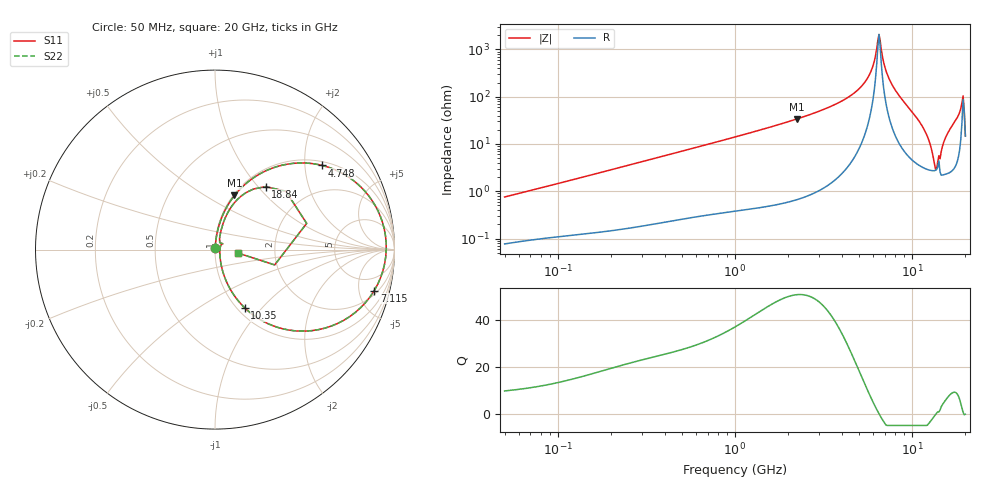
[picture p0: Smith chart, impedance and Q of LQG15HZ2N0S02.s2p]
!Murata Part Number: LQG15HZ2N0S02
!These Parameters are Measured in Series Mode Connection
!  o--[Z]--o
!Port1  Port2
!  o-------o
!Freq. Start=50[MHz] Stop=20[GHz], 401[Steps]
# Hz S RI R 50
!Freq.(Hz) S11(Real) S11(Imag) S21(Real) S21(Imag) S12(Real) S12(Imag) S22(Real) S22(Imag)
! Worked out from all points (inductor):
!   401 points, 50 MHz to 20 GHz, reference 50 ohm
!   read as one part in series: L = 2.36 nH near 51.52 MHz
!   highest Q = 51.1 at 2.245 GHz (marker M1), where L = 2.41 nH
!   self-resonance near 6.503 GHz
!   S11 on the Smith chart (normalised r, x): 50 MHz: 1.00, +0.02; 4.748 GHz: 1.11, +2.45; 7.115 GHz: 2.47, -7.03; 10.35 GHz: 1.08, -0.81; 18.84 GHz: 1.25, +1.10; 20 GHz: 1.29, -0.05
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5e7  0.000824 0.00751  0.9992 -0.00751  0.9992 -0.00751  0.000824 0.00751
1.364002e8  0.00161 0.0196  0.9984 -0.0196  0.9984 -0.0196  0.00161 0.0196
3.721004e8  0.00483 0.0521  0.9952 -0.0521  0.9952 -0.0521  0.00483 0.0521
1e9  0.0229 0.1369  0.9771 -0.1369  0.9771 -0.1369  0.0229 0.1369
2.245319e9  0.1085 0.3014  0.8915 -0.3014  0.8915 -0.3014  0.1085 0.3014
2.728004e9  0.1647 0.3611  0.8353 -0.3611  0.8353 -0.3611  0.1647 0.3611
3.680849e9  0.3263 0.4564  0.6737 -0.4564  0.6737 -0.4564  0.3263 0.4564
4.748272e9  0.597 0.4689  0.403 -0.4689  0.403 -0.4689  0.597 0.4689
5.769027e9  0.8744 0.2746  0.1256 -0.2746  0.1256 -0.2746  0.8744 0.2746
6.503449e9  0.9541 0.00111  0.0459 -0.00111  0.0459 -0.00111  0.9541 0.00111
7.114996e9  0.8871 -0.2287  0.1129 0.2287  0.1129 0.2287  0.8871 -0.2287
7.442007e9  0.8113 -0.3238  0.1887 0.3238  0.1887 0.3238  0.8113 -0.3238
8.644534e9  0.473 -0.4542  0.527 0.4542  0.527 0.4542  0.473 -0.4542
1.034674e10  0.1661 -0.3249  0.8339 0.3249  0.8339 0.3249  0.1661 -0.3249
1.201863e10  0.0521 -0.1489  0.9479 0.1489  0.9479 0.1489  0.0521 -0.1489
1.354865e10  0.027 -0.00939  0.973 0.00939  0.973 0.00939  0.027 -0.00939
1.396067e10  0.0322 0.0249  0.9678 -0.0249  0.9678 -0.0249  0.0322 0.0249
1.550395e10  0.0401 0.1301  0.9599 -0.1301  0.9599 -0.1301  0.0401 0.1301
1.721783e10  0.0939 0.2425  0.9061 -0.2425  0.9061 -0.2425  0.0939 0.2425
1.88369e10  0.2818 0.3509  0.7182 -0.3509  0.7182 -0.3509  0.2818 0.3509
1.912117e10  0.3947 0.3254  0.6053 -0.3254  0.6053 -0.3254  0.3947 0.3254
2e10  0.1286 -0.0194  0.8714 0.0194  0.8714 0.0194  0.1286 -0.0194
